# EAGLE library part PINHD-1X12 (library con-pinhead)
PIN HEADER
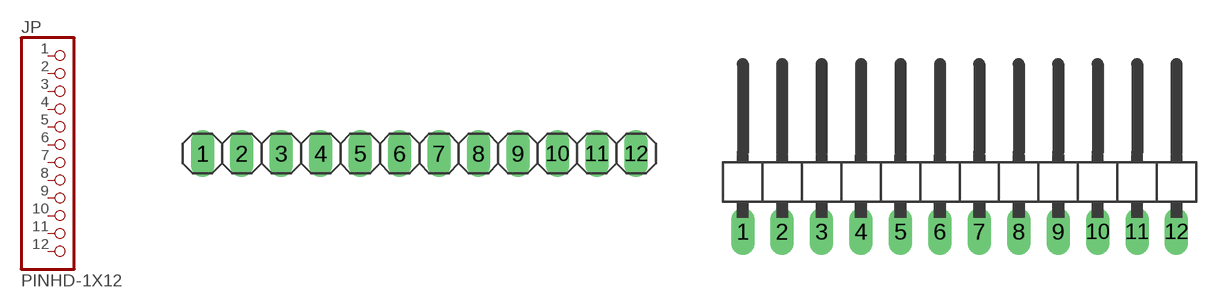
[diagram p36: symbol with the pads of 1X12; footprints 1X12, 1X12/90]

Designator prefix JP

## PINHD-1X12_2.54  [1X12]
1  1  pas
2  2  pas
3  3  pas
4  4  pas
5  5  pas
6  6  pas
7  7  pas
8  8  pas
9  9  pas
10  10  pas
11  11  pas
12  12  pas

## PINHD-1X12_2.54-90°  [1X12/90]
Pads as for 1X12

## PINHD-1X12_2.00  [1X12M]
Pads as for 1X12

## PINHD-1X12_2.54-SMD  [1X12SMD]
Pads as for 1X12

## PINHD-1X12_2.54-SMD-90°  [1X12SMD/90]
Pads as for 1X12

## Footprint 1X12 (pad centres in mm)
PIN HEADER - 2.54
drill 1.016 long: 1 -13.97,0; 2 -11.43,0; 3 -8.89,0; 4 -6.35,0; 5 -3.81,0; 6 -1.27,0; 7 1.27,0; 8 3.81,0; 9 6.35,0; 10 8.89,0; 11 11.43,0; 12 13.97,0

## Footprint 1X12/90 (pad centres in mm)
PIN HEADER - 2.54 90°
drill 1.016 long: 1 -13.97,-3.81; 2 -11.43,-3.81; 3 -8.89,-3.81; 4 -6.35,-3.81; 5 -3.81,-3.81; 6 -1.27,-3.81; 7 1.27,-3.81; 8 3.81,-3.81; 9 6.35,-3.81; 10 8.89,-3.81; 11 11.43,-3.81; 12 13.97,-3.81

## Footprint 1X12M (pad centres in mm)
PIN HEADER - 2
drill 0.914 square: 1 -11,0
drill 0.914: 2 -9,0; 3 -7,0; 4 -5,0; 5 -3,0; 6 -1,0; 7 1,0; 8 3,0; 9 5,0; 10 7,0; 11 9,0; 12 11,0

## Footprint 1X12SMD (pad centres in mm)
PIN HEADER - 2.54 SMD
smd 1.016 x 3.302: 1 -1.27,1.27; 2 1.27,-1.27; 3 3.81,1.27; 4 6.35,-1.27; 5 8.89,1.27; 6 11.43,-1.27; 7 13.97,1.27; 8 16.51,-1.27; 9 19.05,1.27; 10 21.59,-1.27; 11 24.13,1.27; 12 26.67,-1.27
